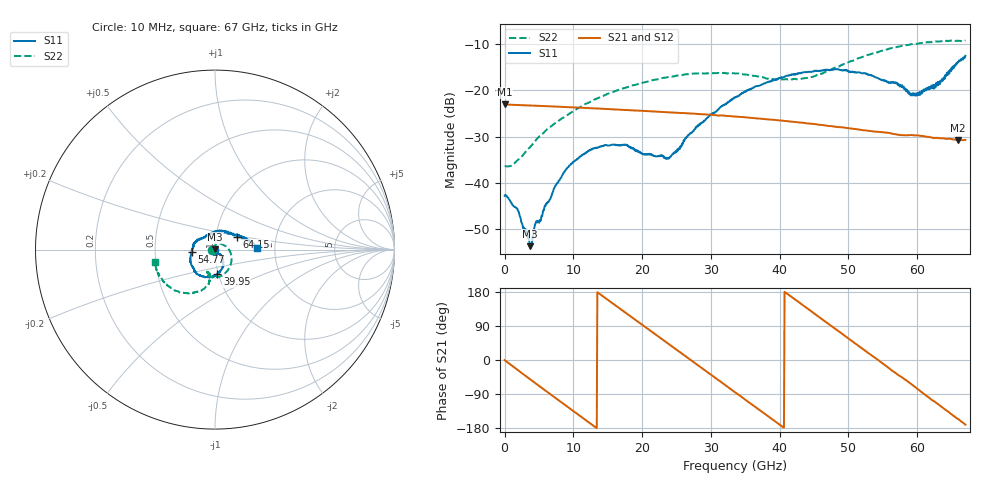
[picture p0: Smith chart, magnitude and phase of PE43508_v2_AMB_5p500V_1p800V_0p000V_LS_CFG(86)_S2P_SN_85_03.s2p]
!Keysight Technologies,N5227A,US51270237,A.10.43.00
!Date: Wednesday, August 22, 2018 17:15:37
!Correction: S11(Full 2 Port(1,3))
!S31(Full 2 Port(1,3))
!S13(Full 2 Port(1,3))
!S33(Full 2 Port(1,3))
!S2P File: Measurements: S11, S31, S13, S33:
# Hz S  dB  R 50
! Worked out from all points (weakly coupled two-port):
!   801 points, 10 MHz to 67 GHz, reference 50 ohm
!   highest |S21| = -23.01 dB at 10 MHz (marker M1); lowest = -30.8 dB at 65.91 GHz (marker M2)
!   lowest |S11| = -53.7 dB at 3.694 GHz (marker M3), VSWR 1.00, Z = 50 + j0.204 ohm
!   |S11| at or under -10 dB: start of sweep to end of sweep
!   |S22| runs from -36.4 to -9.2 dB; largest |S21 - S12| = 0.00035
!   S11 on the Smith chart (normalised r, x): 10 MHz: 0.99, -0.00; 39.95 GHz: 0.99, -0.27; 54.77 GHz: 0.77, -0.02; 64.15 GHz: 1.27, +0.19; 67 GHz: 1.62, +0.03
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1e7  -42.75 -177.4  -23.01 -0.3  -23.01 -0.2  -36.43 -179.7
1.852225e9  -45.57 149.5  -23.14 -25.7  -23.14 -25.7  -35.11 126.0
3.69445e9  -53.65 79.6  -23.25 -50.6  -23.26 -50.6  -32.29 88.5
4.531825e9  -48.72 32.9  -23.30 -61.8  -23.30 -61.8  -30.78 76.0
7.546375e9  -40.34 -32.0  -23.49 -102.2  -23.49 -102.2  -26.87 43.8
9.304862e9  -36.52 -51.2  -23.60 -125.6  -23.60 -125.6  -25.12 27.3
1.123082e10  -33.96 -64.2  -23.74 -151.2  -23.74 -151.1  -23.40 11.2
1.449659e10  -31.91 -83.5  -23.97 165.6  -23.97 165.6  -21.07 -12.0
1.74274e10  -31.78 -94.7  -24.20 127.0  -24.20 127.0  -19.45 -29.8
2.236791e10  -34.15 -82.4  -24.60 61.8  -24.59 61.8  -17.54 -56.3
2.404266e10  -34.38 -65.6  -24.74 39.8  -24.73 39.8  -17.07 -64.0
2.81458e10  -27.75 -42.6  -25.08 -14.2  -25.08 -14.2  -16.29 -81.6
3.3505e10  -21.54 -57.4  -25.64 -85.1  -25.64 -85.1  -16.31 -101.1
3.995279e10  -17.26 -84.6  -26.45 -170.1  -26.46 -170.1  -17.52 -109.1
4.472582e10  -15.94 -107.6  -27.20 126.7  -27.18 126.8  -17.07 -101.2
4.841028e10  -15.40 -126.9  -27.91 77.9  -27.89 77.9  -14.95 -99.7
5.477432e10  -17.71 -173.9  -29.02 -6.4  -28.98 -6.7  -11.41 -116.3
5.586291e10  -18.40 172.9  -29.16 -21.5  -29.15 -21.9  -10.99 -120.4
6.004979e10  -20.50 107.8  -29.70 -76.2  -29.70 -76.7  -9.89 -137.4
6.415292e10  -16.90 30.4  -30.46 -132.1  -30.51 -132.4  -9.30 -155.0
6.591141e10  -13.81 12.4  -30.75 -155.4  -30.82 -155.6  -9.25 -162.4
6.7e10  -12.51 2.0  -30.70 -170.7  -30.79 -170.7  -9.27 -168.3
